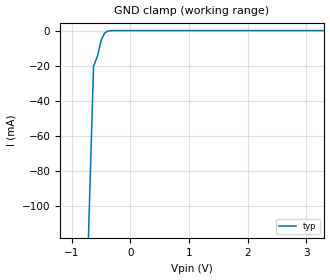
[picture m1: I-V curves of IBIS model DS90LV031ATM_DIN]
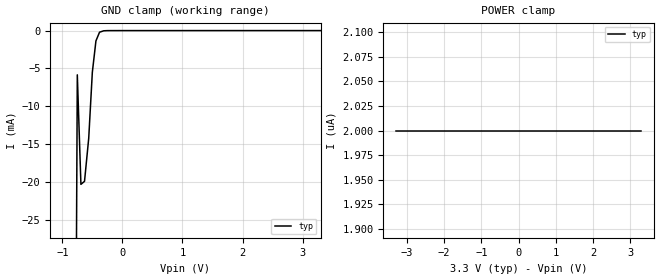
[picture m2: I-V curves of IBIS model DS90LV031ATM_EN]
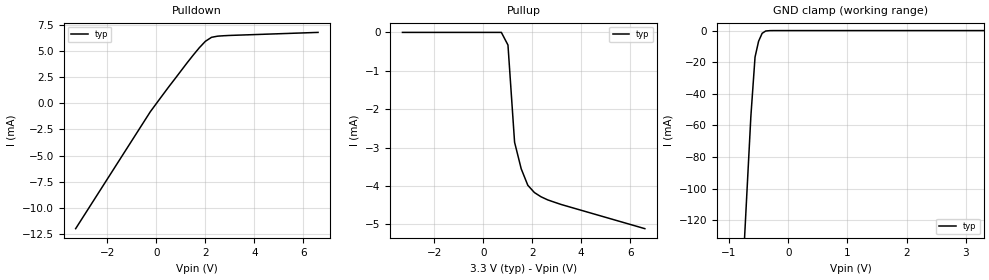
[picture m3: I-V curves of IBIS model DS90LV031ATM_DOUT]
|   National Semiconductor Corporation
|   Interface Products Group
|   IBIS Model of DS90LV031ATM
|   16L SOIC Package
[IBIS Ver]   2.1
[File name]   lv031atm.ibs
[File Rev]   1.2
[Date]   5/30/98
[Source]   File originated at National Semiconductor Corporation.
   Interface Group/Analog Division. All data based on
   Empirical Measurements(Bench).
[Notes]   File created by MS, verified by SBH.
   File Rev 1.2; deleted min/max values from C_comp.
   Reason is typo, should only be typical C_comp---milt
[Disclaimer]
(C) Copyright National Semiconductor Corporation 1994
   All rights reserved
   National Semiconductor Corporation hereby grants
the user of this IBIS model a non-exclusive, nontransferable
license to use this IBIS model under the following terms.
Before using this IBIS model, the user should read this
license.  If the user does not accept these terms,  the
IBIS model should be returned to National within 30 days.
   The user is granted this license only to use the
IBIS model and is not granted rights to sell, load, rent,
lease or license the IBIS model in whole or in part, or in
modified form to anyone other than user. User may modify
the IBIS model to suit its specific applications but rights
to derivative works and such modifications shall belong to
National.
   This IBIS model is provided on an "AS IS" basis and
National makes absolutely no warranty with respect to the
information contained herein.NATIONAL DISCLAIMS AND CUSTOMER
WAIVES ALL WARRANTIES, EXPRESS OR IMPLIED, INCLUDING
WARRANTIES OF MERCHANTABILITY OR FITNESS FOR A PARTICULAR
PURPOSE. The entire risk as to quality and performance is
with the Customer. ACCORDINGLY, IN NO EVENT SHALL THE
COMPANY BE LIABLE FOR ANY DAMAGES, WHETHER IN CONTRACT OR
TORT,INCLUDING ANY LOST PROFITS OR OTHER INCIDENTAL,
CONSEQUENTIAL, EXEMPLARY, OR PUNITIVE DAMAGES ARISING OUT
OF THE USE OR APPLICATION OF THE IBIS model provided in
this package.Further, National reserves the right to make
changes without notice to any product herein to improve
reliability, function, or design. National does not convey
any license under patent rights or any other intellectual
property rights, including those of third parties.
   National is not obligated to provide maintenance or support
for the licensed IBIS model.
Contact National at ATTN:INTERFACE APPLICATIONS/IBIS MODELS.
2900 Semiconductor Drive, M/S A2595, Santa Clara, CA 95052-8090
[Copyright]   Copyright 1994, National Semiconductor, All Rights Reserved
[Component]   DS90LV031ATM
[Manufacturer]  National Semiconductor Corp
[Package]
|   typ   min   max
R_pkg   50.0m   NA   NA
L_pkg   1.37nH   NA   NA
C_pkg   0.26pF   NA   NA
[Pin]   signal_name   model_name   R_pin   L_pin   C_pin
1   DIN1   DS90LV031ATM_DIN   50.0m   2.07n   0.429p
2   DOUT1+   DS90LV031ATM_DOUT   50.0m   1.49n   0.306p
3   DOUT1-   DS90LV031ATM_DOUT   50.0m   0.95n   0.146p
4   EN   DS90LV031ATM_EN   50.0m   0.95n   0.152p
5   DOUT2-   DS90LV031ATM_DOUT   50.0m   0.95n   0.152p
6   DOUT2+   DS90LV031ATM_DOUT   50.0m   0.95n   0.146p
7   DIN2   DS90LV031ATM_DIN   50.0m   1.49n   0.306p
8   GND   GND   50.0m   2.07n   0.429p
9   DIN3   DS90LV031ATM_DIN   50.0m   2.07n   0.429p
10   DOUT3+   DS90LV031ATM_DOUT   50.0m   1.49n   0.306p
11   DOUT3-   DS90LV031ATM_DOUT   50.0m   0.95n   0.146p
12   EN*   DS90LV031ATM_EN   50.0m   0.95n   0.152p
13   DOUT4-   DS90LV031ATM_DOUT   50.0m   0.95n   0.152p
14   DOUT4+   DS90LV031ATM_DOUT   50.0m   0.95n   0.146p
15   DIN4   DS90LV031ATM_DIN   50.0m   1.49n   0.306p
16   VCC   POWER   50.0m   2.07n   0.429p
[Diff_pin]   inv_pin   vdiff   tdelay_typ   tdelay_min   tdelay_max
| The '+' pin is Diff_pin and the '-' pin is the inv_pin
2   3   NA   0 0 0
6   5   NA   0 0 0
10   11   NA   0 0 0
14   13   NA   0 0 0
| Models and submodels in the file (3): DS90LV031ATM_DIN (Input), DS90LV031ATM_EN (Input), DS90LV031ATM_DOUT (3-state)
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|   Driver Input  MODEL
[Model]   DS90LV031ATM_DIN
Model_type   Input
|Signals   DIN1,DIN2,DIN3,DIN4
Vinh = 2.0
Vinl = 0.8
|   typ   min   max
C_comp   2.757pF   NA   NA
|   typ   min   max
[Temperature Range]   25.0   NA   NA
[Voltage range]   3.3V   3.0V   3.6V
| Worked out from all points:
|   GND clamp passes 1 mA (typ) near -0.42 V on its own axis
[Power_clamp]
| Note that the[POWER_clamp]voltage table is referenced to Vcc
| and is calculated using Vtable=Vcc - Vmeasured.
| Driver Inputs do not have Power Clamp
| Voltage   I(typ)   I(min)   I(max)
-3.3V     0A         NA         NA
3.3V      0A         NA         NA
[GND_clamp]
|Voltage   I(typ)   I(min)   I(max)
-3.3V     -3.01A     NA         NA
-690mV    -87.5mA    NA         NA
-630mV    -20.4mA    NA         NA
-560mV    -14.2mA    NA         NA
-500mV    -5.5mA     NA         NA
-440mV    -1.37mA    NA         NA
-380mV    -214uA     NA         NA
3.3V      0A         NA         NA
|   Driver Enable  MODEL
[Model]   DS90LV031ATM_EN
Model_type   Input
|Signals   EN,EN*
Vinh = 2.0
Vinl = 0.8
|   typ   min   max
C_comp   2.757pF   NA   NA
|   typ   min   max
[Temperature Range]   25.0   NA   NA
[Voltage range]   3.3V   3.0V   3.6V
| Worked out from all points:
|   GND clamp passes 1 mA (typ) near -0.42 V on its own axis
[GND_clamp]
|Voltage   I(typ)   I(min)   I(max)
-3.3V     -4.01A     NA         NA
-750mV    -5.84mA    NA         NA
-690mV    -20.3mA    NA         NA
-630mV    -19.9mA    NA         NA
-560mV    -14.2mA    NA         NA
-500mV    -5.51mA    NA         NA
-440mV    -1.36mA    NA         NA
-380mV    -212uA     NA         NA
-250mV    -4.56uA    NA         NA
3.3V      2uA        NA         NA
[Power_clamp]
| Note that the[POWER_clamp]voltage table is referenced to Vcc
| and is calculated using Vtable=Vcc - Vmeasured.
| Enble Inputs (EN,EN*) have no Power Clamp
| Voltage   I(typ)   I(min)   I(max)
-3.3V     2uA        NA         NA
3.3V      2uA        NA         NA
|   Driver Output  MODEL
[Model]   DS90LV031ATM_DOUT
Model_type   3-state
| Signals   DOUT1+,DOUT1-,DOUT2+,DOUT2-,DOUT3+,DOUT3-,DOUT4+,DOUT4-
Vmeas = 1.2V   |This is 0.0v differential on ouput
Cref = 5pF   |Timing specification test load capacitance value
Rref = 50   |Note: 100 Ohm between the two driver outputs
Vref = 1.2   |Timing specification test load voltage; GND
| variable   typ   min   max
C_comp   3.750pF   NA   NA
|   typ   min   max
[Temperature Range]   25.0   NA   NA
[Voltage range]   3.3V   3.0V   3.6V
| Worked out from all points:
|   slope of the pulldown table from 0 to 0.495 V, typ, clamps not added: 317 ohm
|   GND clamp passes 1 mA (typ) near -0.41 V on its own axis
[Pulldown]
| Voltage   I(typ)   I(min)   I(max)
-3.3V     -12mA      NA         NA
-250mV    -804uA     NA         NA
1.25V     3.87mA     NA         NA
1.75V     5.32mA     NA         NA
2V        5.94mA     NA         NA
2.25V     6.32mA     NA         NA
2.5V      6.43mA     NA         NA
6.6V      6.79mA     NA         NA
[Pullup]
| Note that the[Pullup]voltage table is referenced to Vcc
| and is calculated using Vtable=Vcc - Vmeasured.
| Driver Outputs do not have Power Clamp
|  Voltage   I(typ)   I(min)   I(max)
-3.3V     729pA      NA         NA
740mV     -86.1nA    NA         NA
1.01V     -329uA     NA         NA
1.28V     -2.86mA    NA         NA
1.55V     -3.55mA    NA         NA
1.82V     -3.98mA    NA         NA
2.09V     -4.17mA    NA         NA
2.63V     -4.36mA    NA         NA
3.18V     -4.48mA    NA         NA
6.6V      -5.11mA    NA         NA
[GND_clamp]
| Outputs in Tri-state.
|  Voltage   I(typ)   I(min)   I(max)
-3.3V     -1.99A     NA         NA
-690mV    -97.3mA    NA         NA
-630mV    -54.1mA    NA         NA
-560mV    -16.8mA    NA         NA
-500mV    -6.75mA    NA         NA
-440mV    -1.73mA    NA         NA
-380mV    -271uA     NA         NA
3.3V      0A         NA         NA
[POWER_clamp]
| Note that the[POWER_clamp]voltage table is referenced to Vcc
| and is calculated using Vtable=Vcc - Vmeasured.
| Outputs in Tri-state.
| No Power Clamp in Tri-State
|  Voltage   I(typ)   I(min)   I(max)
-3.3V     0A         NA         NA
3.3V      0A         NA         NA
[Ramp]
| Note: Ramp rate measured on single-ended Driver Output.
|   typ   min   max
dV/dt_r   0.183/350.0p   NA   NA
dV/dt_f   0.200/330.0p   NA   NA
R_load = 100Ohm | Note: This 100 Ohm is across the two driver output
